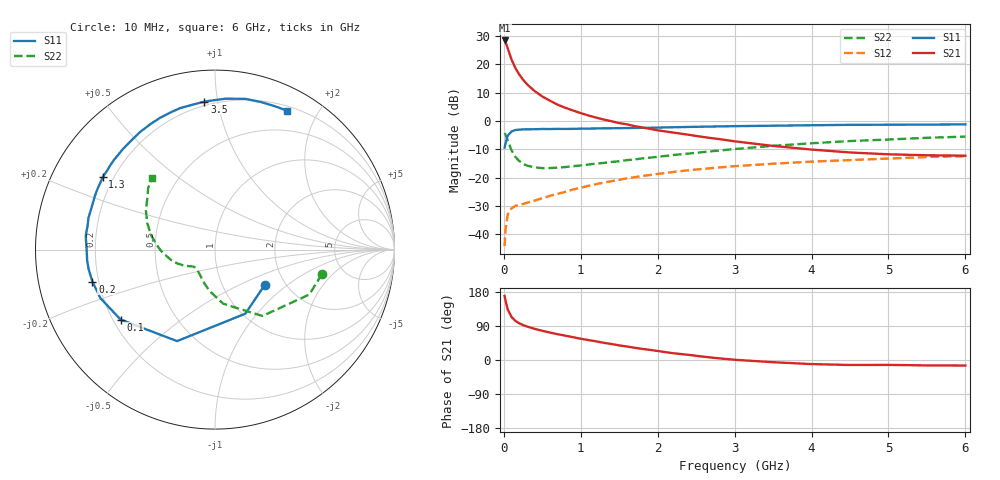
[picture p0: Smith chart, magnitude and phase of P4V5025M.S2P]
! SIEMENS Small Signal Semiconductors
! BFP182
! Si NPN RF Bipolar Junction Transistor in SOT143
! VCE = 0.5 V  IC = 25 mA
! Common Emitter S-Parameters:  March  1996
# GHz  S  MA  R  50
!  f  S11  S21  S12  S22
! GHz  MAG  ANG  MAG  ANG  MAG  ANG  MAG  ANG
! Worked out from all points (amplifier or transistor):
!   36 points, 10 MHz to 6 GHz, reference 50 ohm
!   highest |S21| = 28.4 dB at 10 MHz (marker M1)
!   |S21| within 3 dB of that: start of sweep to 53.13 MHz
!   unconditionally stable (mu >= 1): start of sweep to 18.55 MHz; 174.9 MHz to end of sweep
!   at 250 MHz: K = 1.31, MAG = 18.6 dB, |S12| = -29.3 dB
!   at 1.4 GHz: K = 2.55, MAG = 3.7 dB, |S12| = -21.2 dB
!   at 6 GHz: K = 1.90, MAG = -5.4 dB, |S12| = -12.4 dB
!   S11 on the Smith chart (normalised r, x): 10 MHz: 1.57, -0.70; 100 MHz: 0.23, -0.31; 200 MHz: 0.18, -0.12; 1.3 GHz: 0.16, +0.29; 3.5 GHz: 0.18, +0.92; 6 GHz: 0.25, +1.62
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0.01  0.3399 -35.7  26.4 168.8  0.0062 72.4  0.6116 -12.9
0.02  0.3949 -64.6  25.28 158.1  0.0117 67.7  0.5818 -25.5
0.05  0.552 -112.5  19.24 133.7  0.0225 49.5  0.4543 -54.5
0.1  0.6548 -143.5  12.15 113.5  0.0288 35.0  0.3049 -81.4
0.15  0.6934 -157.1  8.619 103.2  0.0319 31.7  0.233 -97.3
0.2  0.706 -165.4  6.624 96.8  0.033 32.0  0.1968 -107.7
0.25  0.7125 -171.2  5.352 92.1  0.0344 32.5  0.176 -115.1
0.3  0.7149 -175.0  4.472 88.4  0.0362 34.5  0.1635 -120.9
0.4  0.7162 178.8  3.385 82.2  0.0394 37.7  0.1523 -129.3
0.5  0.7245 173.8  2.716 77.1  0.0436 40.3  0.1478 -134.3
0.6  0.7221 169.5  2.28 72.4  0.0479 42.9  0.148 -137.3
0.7  0.727 165.8  1.942 68.0  0.0521 45.2  0.1507 -139.8
0.9  0.7277 159.6  1.532 60.3  0.0621 47.5  0.1598 -144.1
1.1  0.7368 152.7  1.253 52.6  0.0721 48.3  0.1708 -147.0
1.3  0.7445 147.2  1.061 45.3  0.082 48.2  0.1825 -150.3
1.7  0.7551 135.4  0.814 32.3  0.1023 46.0  0.2101 -157.2
2.2  0.7767 122.6  0.626 17.9  0.126 41.6  0.2513 -166.6
2.8  0.8033 108.0  0.48 4.3  0.1517 35.0  0.3018 -179.0
3.5  0.827 94.1  0.364 -5.8  0.1766 26.8  0.3649 167.3
4.5  0.8566 78.7  0.279 -13.1  0.205 15.8  0.4435 150.3
5.5  0.8653 67.6  0.249 -14.3  0.2321 5.9  0.5064 137.3
6  0.8726 62.5  0.245 -14.6  0.2399 0.3  0.5309 131.2
